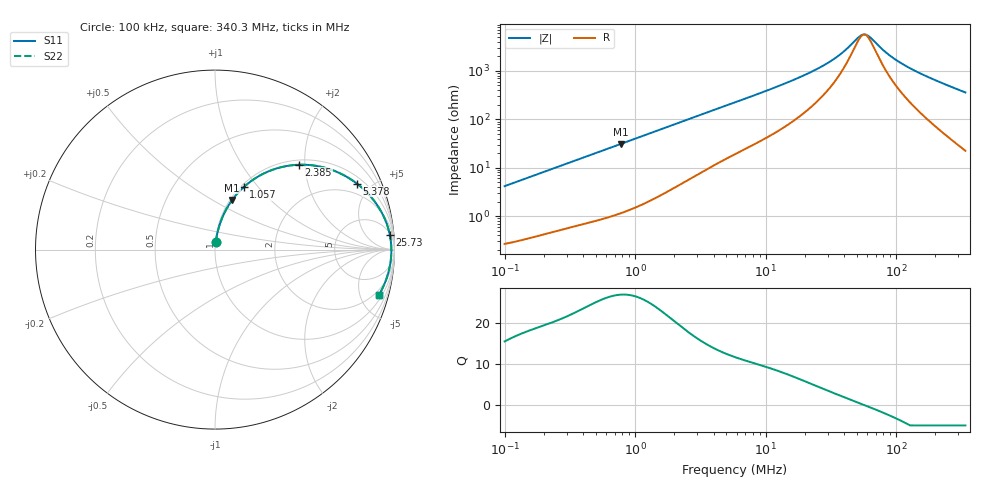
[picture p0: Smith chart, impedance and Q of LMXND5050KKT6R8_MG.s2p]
! LMXND5050KKT6R8_MG  S-PARAMETER MODEL  ( General Type )
! Model Generated by TAIYO YUDEN Corporation (http://www.ty-top.com)
! Version 1.0
! TAIYO YUDEN Control No. 191023NI43SB-FBB
! Copyright(c) 2019 TAIYO YUDEN CO.,LTD. All Rights Reserved.
! Product Description (link to TY-COMPAS)
! https://ds.yuden.co.jp/TYCOMPAS/or/detail?pn=LMXND5050KKT6R8MMG&u=M
! Products Name : Inductors
! Characteristics :
!  Inductance : 6.8 uH , SRF(min) : 33 MHz , DC Resistance(max) : 0.222 Ohm
!  Rated Current : Saturation :1000 mA , Temp Rise : 1000 mA
!  Case Size : 4.9 x 4.9 / 0.193 x 0.193 [mm/inch] , Thickness : 1 / 0.039 [mm/inch]
!  (Conditions: Temperature = 25 degC , DC Bias Current/Voltage = 0A / 0V)
! External Node Assignments :
!  1  o---GGG---o  2
! GND o---------o GND
! Frequency Range : 0.1MHz  -  340.31115MHz  [ 402 STEP ]
# MHz S RI R 50
! Freq[MHz].  S11 Real  S11 Imag  S21 Real  S21 Imag  S12 Real  S12 Imag  S22 Real  S22 Imag
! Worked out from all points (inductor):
!   401 points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, 100 kHz to 340.3 MHz, reference 50 ohm
!   read as one part in series: L = 6.57 uH near 104.2 kHz
!   highest Q = 27.1 at 779.5 kHz (marker M1), where L = 6.34 uH
!   self-resonance near 57.08 MHz
!   S11 on the Smith chart (normalised r, x): 100 kHz: 1.01, +0.08; 1.057 MHz: 1.03, +0.84; 2.385 MHz: 1.10, +1.87; 5.378 MHz: 1.34, +4.12; 25.73 MHz: 6, +22; 340.3 MHz: 1.45, -7.15
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0.1  0.00435 0.0411  0.9957 -0.0411  0.9957 -0.0411  0.00435 0.0411
0.207907  0.0114 0.0836  0.9886 -0.0836  0.9886 -0.0836  0.0114 0.0836
0.390471  0.0303 0.1513  0.9697 -0.1513  0.9697 -0.1513  0.0303 0.1513
0.779469  0.0964 0.2772  0.9036 -0.2772  0.9036 -0.2772  0.0964 0.2772
1.057412  0.1591 0.3473  0.8409 -0.3473  0.8409 -0.3473  0.1591 0.3473
1.524679  0.2752 0.4258  0.7248 -0.4258  0.7248 -0.4258  0.2752 0.4258
2.384689  0.469 0.4729  0.531 -0.4729  0.531 -0.4729  0.469 0.4729
3.438477  0.6334 0.4499  0.3666 -0.4499  0.3666 -0.4499  0.6334 0.4499
5.377982  0.7915 0.3672  0.2085 -0.3672  0.2085 -0.3672  0.7915 0.3672
5.953437  0.8188 0.3446  0.1812 -0.3446  0.1812 -0.3446  0.8188 0.3446
10.73566  0.923 0.2172  0.077 -0.2172  0.077 -0.2172  0.923 0.2172
22.77862  0.9711 0.0959  0.0289 -0.0959  0.0289 -0.0959  0.9711 0.0959
25.73389  0.9744 0.0808  0.0256 -0.0808  0.0256 -0.0808  0.9744 0.0808
36.35886  0.9802 0.043  0.0198 -0.043  0.0198 -0.043  0.9802 0.043
51.37064  0.9825 0.00977  0.0175 -0.00977  0.0175 -0.00977  0.9825 0.00977
55.7229  0.9826 0.00222  0.0174 -0.00222  0.0174 -0.00222  0.9826 0.00222
59.22742  0.9827 -0.00344  0.0173 0.00344  0.0173 0.00344  0.9827 -0.00344
62.95234  0.9826 -0.00911  0.0174 0.00911  0.0174 0.00911  0.9826 -0.00911
88.94399  0.981 -0.0425  0.019 0.0425  0.019 0.0425  0.981 -0.0425
113.5201  0.9781 -0.0686  0.0219 0.0686  0.0219 0.0686  0.9781 -0.0686
150.8998  0.9718 -0.104  0.0282 0.104  0.0282 0.104  0.9718 -0.104
340.3111  0.9144 -0.2503  0.0856 0.2503  0.0856 0.2503  0.9144 -0.2503
